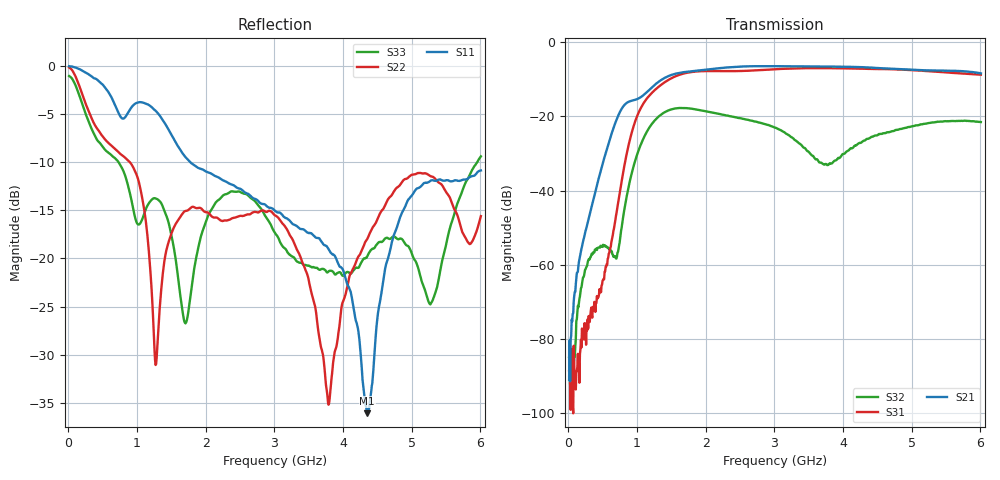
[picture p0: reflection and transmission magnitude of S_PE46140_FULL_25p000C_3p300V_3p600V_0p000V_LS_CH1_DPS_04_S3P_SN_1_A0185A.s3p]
! Device ID: PE46140_FULL
! File Path: z:\PE46140\MajorStates\25p000C\3p300\LS_CH1_DPS_04\PE46140_FULL_25p000C_3p300V_3p600V_0p000V_LS_CH1_DPS_04_S3P_SN_1_A0185A.s3p
! Serial: 1
! Lot: A0185A
! Temp: 25.000C
! VDD: 3.300
! VSS: 0.000
! Control_Hi: 3.600
! Control_Lo: 0.000
! Logic State: LS_CH1_DPS_04
! Port 1: RFIN
! Port 2: RFOUT1
! Port 3: RFOUT2
! ThroughPath:1-2
! IDD: 0.0003112086
! ISS: -1.694e-007
! Comment:
#  Hz  S  RI  R  50
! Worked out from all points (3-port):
!   801 points, 10 MHz to 6.01 GHz, reference 50 ohm
!   strongest paths, dB at 10 MHz, 1.51 GHz, 3.01 GHz, 4.51 GHz, 6.01 GHz:
!     S21: -91.0, -8.8, -6.5, -7.0, -8.4
!     S31: -88.7, -9.7, -7.3, -7.3, -8.8
!     S32: -85.0, -18.1, -23.1, -25.0, -21.6
!   lowest |S11| = -36.1 dB at 4.353 GHz (marker M1), VSWR 1.03, Z = 48.5 + j0.434 ohm
!   |S11| at or under -10 dB: 1.772 GHz to end of sweep
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1e7  0.9924 -0.0707  1.26e-05 3.76e-05  3.66e-05 1.68e-05
     2.7e-05 8.11e-06  0.9748 -0.0927  -7.19e-06 5.73e-05
     5.2e-06 -3.62e-05  4.34e-05 3.54e-05  0.8808 -0.083
3.325e8  -0.3244 -0.8235  -0.00572 0.000754  -3.29e-05 0.000208
         -0.00572 0.000764  -0.4381 -0.3155  -0.000442 0.00129
         -9.3e-05 0.000249  -0.000427 0.00127  -0.3865 -0.2764
8.05e8  -0.5296 -0.0577  -0.0144 0.1374  0.0187 -0.00407
        -0.0146 0.1374  0.1127 0.3191  -0.00112 0.00473
        0.0187 -0.00411  -0.00112 0.0047  0.1024 0.2629
1.3975e9  -0.3504 0.3685  0.3146 -0.0876  -0.1512 0.2412
          0.3151 -0.0872  -0.0198 0.0945  -0.0648 0.092
          -0.1516 0.2414  -0.0649 0.0921  0.16 -0.0764
1.975e9  -0.1283 0.257  -0.1592 -0.3891  0.401 -0.0568
         -0.1592 -0.3896  0.1619 0.0678  0.0372 -0.1121
         0.4015 -0.0567  0.0372 -0.1122  0.0515 0.1362
3.01e9  0.00703 0.1766  -0.1553 0.4459  -0.3727 -0.2126
        -0.156 0.4458  0.1496 -0.0748  0.0466 0.0525
        -0.3731 -0.2129  0.0468 0.0524  0.1264 -0.0498
3.79e9  -0.0121 0.1112  0.4504 0.1226  -0.2095 0.3914
        0.4503 0.1231  0.0164 -0.00575  -0.0224 -0.000165
        -0.2095 0.3912  -0.0223 -0.000288  0.083 -0.0217
4.3525e9  -0.0151 0.00448  0.2789 -0.3594  0.2408 0.3621
          0.2797 -0.3589  0.1023 0.0733  0.0487 0.00958
          0.2415 0.3621  0.0488 0.00956  0.0984 -0.0275
4.9225e9  -0.1178 -0.1515  -0.2071 -0.3719  0.4203 -0.0342
          -0.2069 -0.3728  0.2571 0.0296  -0.0339 -0.0612
          0.4212 -0.0338  -0.0338 -0.0613  0.0908 -0.0742
6.01e9  -0.2324 -0.1669  -0.0919 0.3667  -0.1625 -0.3231
        -0.0921 0.3669  0.1558 0.0568  0.0586 0.0593
        -0.1641 -0.3238  0.059 0.0593  0.3163 0.121
